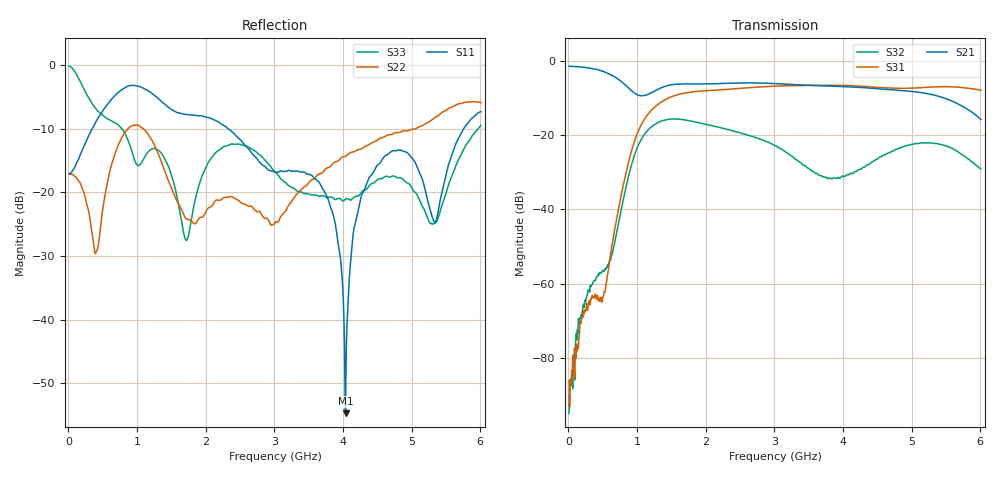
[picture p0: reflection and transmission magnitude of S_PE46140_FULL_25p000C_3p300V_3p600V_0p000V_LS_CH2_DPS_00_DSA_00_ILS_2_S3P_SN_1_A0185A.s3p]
! Device ID: PE46140_FULL
! File Path: z:\PE46140\MajorStates\25p000C\3p300\LS_CH2_DPS_00_DSA_00_ILS_2\PE46140_FULL_25p000C_3p300V_3p600V_0p000V_LS_CH2_DPS_00_DSA_00_ILS_2_S3P_SN_1_A0185A.s3p
! Serial: 1
! Lot: A0185A
! Temp: 25.000C
! VDD: 3.300
! VSS: 0.000
! Control_Hi: 3.600
! Control_Lo: 0.000
! Logic State: LS_CH2_DPS_00_DSA_00_ILS_2
! Port 1: RFIN
! Port 2: RFOUT1
! Port 3: RFOUT2
! ThroughPath:1-3
! IDD: 0.0003146857
! ISS: -1.794e-007
! Comment:
#  Hz  S  RI  R  50
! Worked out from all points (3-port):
!   801 points, 10 MHz to 6.01 GHz, reference 50 ohm
!   strongest paths, dB at 10 MHz, 1.51 GHz, 3.01 GHz, 4.51 GHz, 6.01 GHz:
!     S21: -1.5, -6.5, -6.2, -7.6, -15.8
!     S31: -86.0, -9.6, -6.9, -7.2, -8.0
!     S32: -94.8, -15.7, -22.9, -26.2, -29.1
!   lowest |S11| = -54.7 dB at 4.037 GHz (marker M1), VSWR 1.00, Z = 50.1 - j0.167 ohm
!   |S11| at or under -10 dB: start of sweep to 346.1 MHz; 2.326 GHz to 5.759 GHz (3.434 GHz wide, 84.9 % of centre)
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1e7  0.14 -0.0109  0.842 -0.0244  4.51e-06 -5.9e-05
     0.8417 -0.0242  0.1399 -0.00673  -2.73e-05 -2.2e-05
     3.79e-05 -3.3e-05  -5.99e-06 -1.72e-05  0.9744 -0.0929
3.55e8  -0.0161 -0.3218  0.4591 -0.6282  -0.000522 -0.000262
        0.4593 -0.6262  -0.00908 -0.0426  -0.00013 0.00101
        -0.000618 -0.000263  -0.000155 0.00102  -0.4312 -0.2281
1.165e9  -0.5849 0.2243  -0.2046 -0.288  -0.1908 -0.0291
         -0.2047 -0.2887  0.2131 -0.1872  -0.00331 0.1182
         -0.1911 -0.0294  -0.00342 0.1181  0.1811 0.1039
1.9825e9  -0.1827 0.3481  -0.4184 0.2469  0.3882 -0.0567
          -0.4186 0.2468  0.0622 -0.0256  -0.1398 -0.0176
          0.3884 -0.0564  -0.1397 -0.0178  0.0498 0.1401
3.01e9  0.0156 0.1431  0.4091 0.2714  -0.3905 -0.2305
        0.4088 0.2724  -0.0576 -0.0013  0.0646 -0.0318
        -0.3908 -0.2312  0.0646 -0.0319  0.1317 -0.0598
3.7675e9  0.0284 0.0884  0.2754 -0.3639  -0.2442 0.3967
          0.2762 -0.3634  0.0773 0.1346  -0.0148 0.0217
          -0.2446 0.3965  -0.0147 0.0217  0.0851 -0.0302
4.0375e9  0.000788 -0.00167  0.0428 -0.443  -0.009 0.4631
          0.0434 -0.4434  0.1394 0.1324  0.0238 0.0156
          -0.00858 0.4627  0.0238 0.0154  0.0826 -0.0316
4.3825e9  -0.1038 -0.0794  -0.2532 -0.3445  0.2675 0.3566
          -0.2532 -0.3452  0.2158 0.099  0.0155 -0.0375
          0.2676 0.3563  0.0152 -0.0374  0.1044 -0.0426
5.3425e9  -0.0399 -0.0424  -0.1019 0.3252  0.3236 -0.3045
          -0.1029 0.3255  0.3853 -0.0395  0.0131 0.0758
          0.3234 -0.3042  0.0132 0.0761  0.0574 0.00389
6.01e9  -0.2933 -0.3141  0.1534 0.0485  -0.2002 -0.3446
        0.1541 0.0488  0.2469 -0.4429  0.0292 -0.019
        -0.2013 -0.3455  0.0293 -0.0191  0.3059 0.1365
